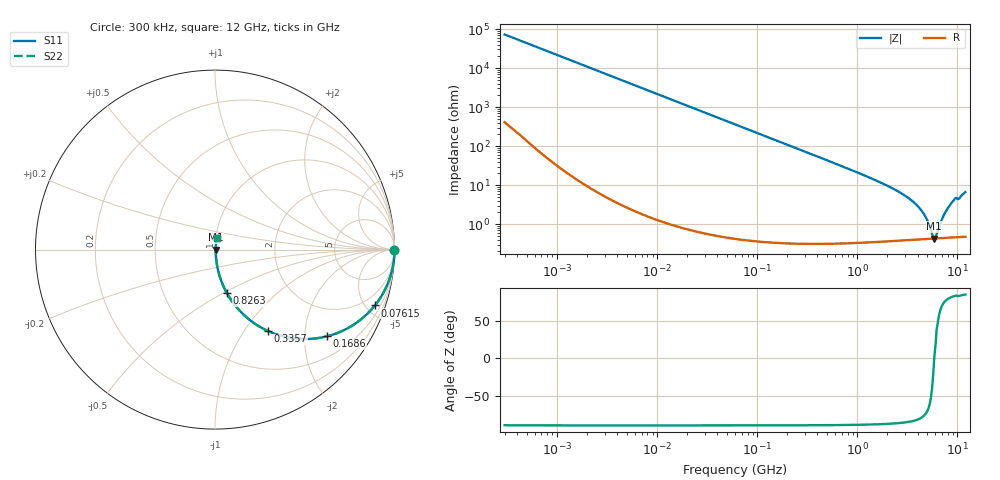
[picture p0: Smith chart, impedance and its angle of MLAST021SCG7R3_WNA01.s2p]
! MLAST021SCG7R3_WNA01  S-PARAMETER MODEL  ( General Type )
! Model Generated by TAIYO YUDEN Corporation (http://www.ty-top.com)
! Version 1.0
! TAIYO YUDEN Control No. 220901
! Copyright(c) 2022 TAIYO YUDEN CO.,LTD. All Rights Reserved.
! Product Description (link to TY-COMPAS)
! https://ds.yuden.co.jp/TYCOMPAS/or/detail?pn=MLAST021SCG7R3CWNA01&u=M
! Products Name : Multilayer Ceramic Capacitors
! Characteristics :
!  Capacitance : 7.3 pF , Rated Voltage : 25V , TCC : CG / C0G
!  Case Size : 0.25 x 0.125 / 0.0098 x 0.0049 [mm/inch] , Thickness : 0.125 / 0.0049 [mm/inch]
!  (Conditions: Temperature = 25 degC , DC Bias Current/Voltage = 0A / 0V)
! External Node Assignments :
!  1  o---| |---o  2
! GND o---------o GND
! Frequency Range : 0.3MHz  -  12000MHz  [ 401 STEP ]
# MHz S RI R 50
! Freq[MHz].  S11 Real  S11 Imag  S21 Real  S21 Imag  S12 Real  S12 Imag  S22 Real  S22 Imag
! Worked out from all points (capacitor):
!   401 points, 300 kHz to 12 GHz, reference 50 ohm
!   read as one part in series: C = 7.3 pF near 316.3 kHz
!   lowest |Z| = 430 mohm at 5.869 GHz (marker M1)
!   series resonance near 5.859 GHz, so ESL is about 100 pH
!   S11 on the Smith chart (normalised r, x): 300 kHz: open; 76.15 MHz: 1.01, -5.72; 168.6 MHz: 1.01, -2.58; 335.7 MHz: 1.01, -1.29; 826.3 MHz: 1.01, -0.52; 12 GHz: 1.01, +0.13
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0.3  1 -0.00138  9.65e-06 0.00138  9.65e-06 0.00138  1 -0.00138
1.769972  0.9999 -0.00812  7.34e-05 0.00812  7.34e-05 0.00812  0.9999 -0.00812
10.44266  0.9977 -0.0478  0.00232 0.0478  0.00232 0.0478  0.9977 -0.0478
27.10171  0.9847 -0.1224  0.0153 0.1224  0.0153 0.1224  0.9847 -0.1224
60  0.9293 -0.2557  0.0707 0.2557  0.0707 0.2557  0.9293 -0.2557
76.15486  0.8909 -0.3111  0.1091 0.3111  0.1091 0.3111  0.8909 -0.3111
168.5979  0.6251 -0.4828  0.3749 0.4828  0.3749 0.4828  0.6251 -0.4828
335.7268  0.2962 -0.4542  0.7038 0.4542  0.7038 0.4542  0.2962 -0.4542
353.9943  0.2746 -0.4438  0.7254 0.4438  0.7254 0.4438  0.2746 -0.4438
526.7124  0.1462 -0.3495  0.8538 0.3495  0.8538 0.3495  0.1462 -0.3495
826.3444  0.0653 -0.2409  0.9347 0.2409  0.9347 0.2409  0.0653 -0.2409
2088.533  0.0118 -0.0897  0.9882 0.0897  0.9882 0.0897  0.0118 -0.0897
3107.553  0.00638 -0.0499  0.9936 0.0499  0.9936 0.0499  0.00638 -0.0499
4050.141  0.00482 -0.0278  0.9952 0.0278  0.9952 0.0278  0.00482 -0.0278
4747.894  0.00439 -0.0156  0.9956 0.0156  0.9956 0.0156  0.00439 -0.0156
5565.855  0.00426 -0.00372  0.9957 0.00372  0.9957 0.00372  0.00426 -0.00372
5868.704  0.00428 0.000121  0.9957 -0.000121  0.9957 -0.000121  0.00428 0.000121
6188.031  0.00433 0.00342  0.9957 -0.00342  0.9957 -0.00342  0.00433 0.00342
7254.098  0.00467 0.0157  0.9953 -0.0157  0.9953 -0.0157  0.00467 0.0157
8503.825  0.00552 0.0315  0.9945 -0.0315  0.9945 -0.0315  0.00552 0.0315
9207.246  0.00622 0.0405  0.9938 -0.0405  0.9938 -0.0405  0.00622 0.0405
12000  0.00906 0.0654  0.9909 -0.0654  0.9909 -0.0654  0.00906 0.0654
